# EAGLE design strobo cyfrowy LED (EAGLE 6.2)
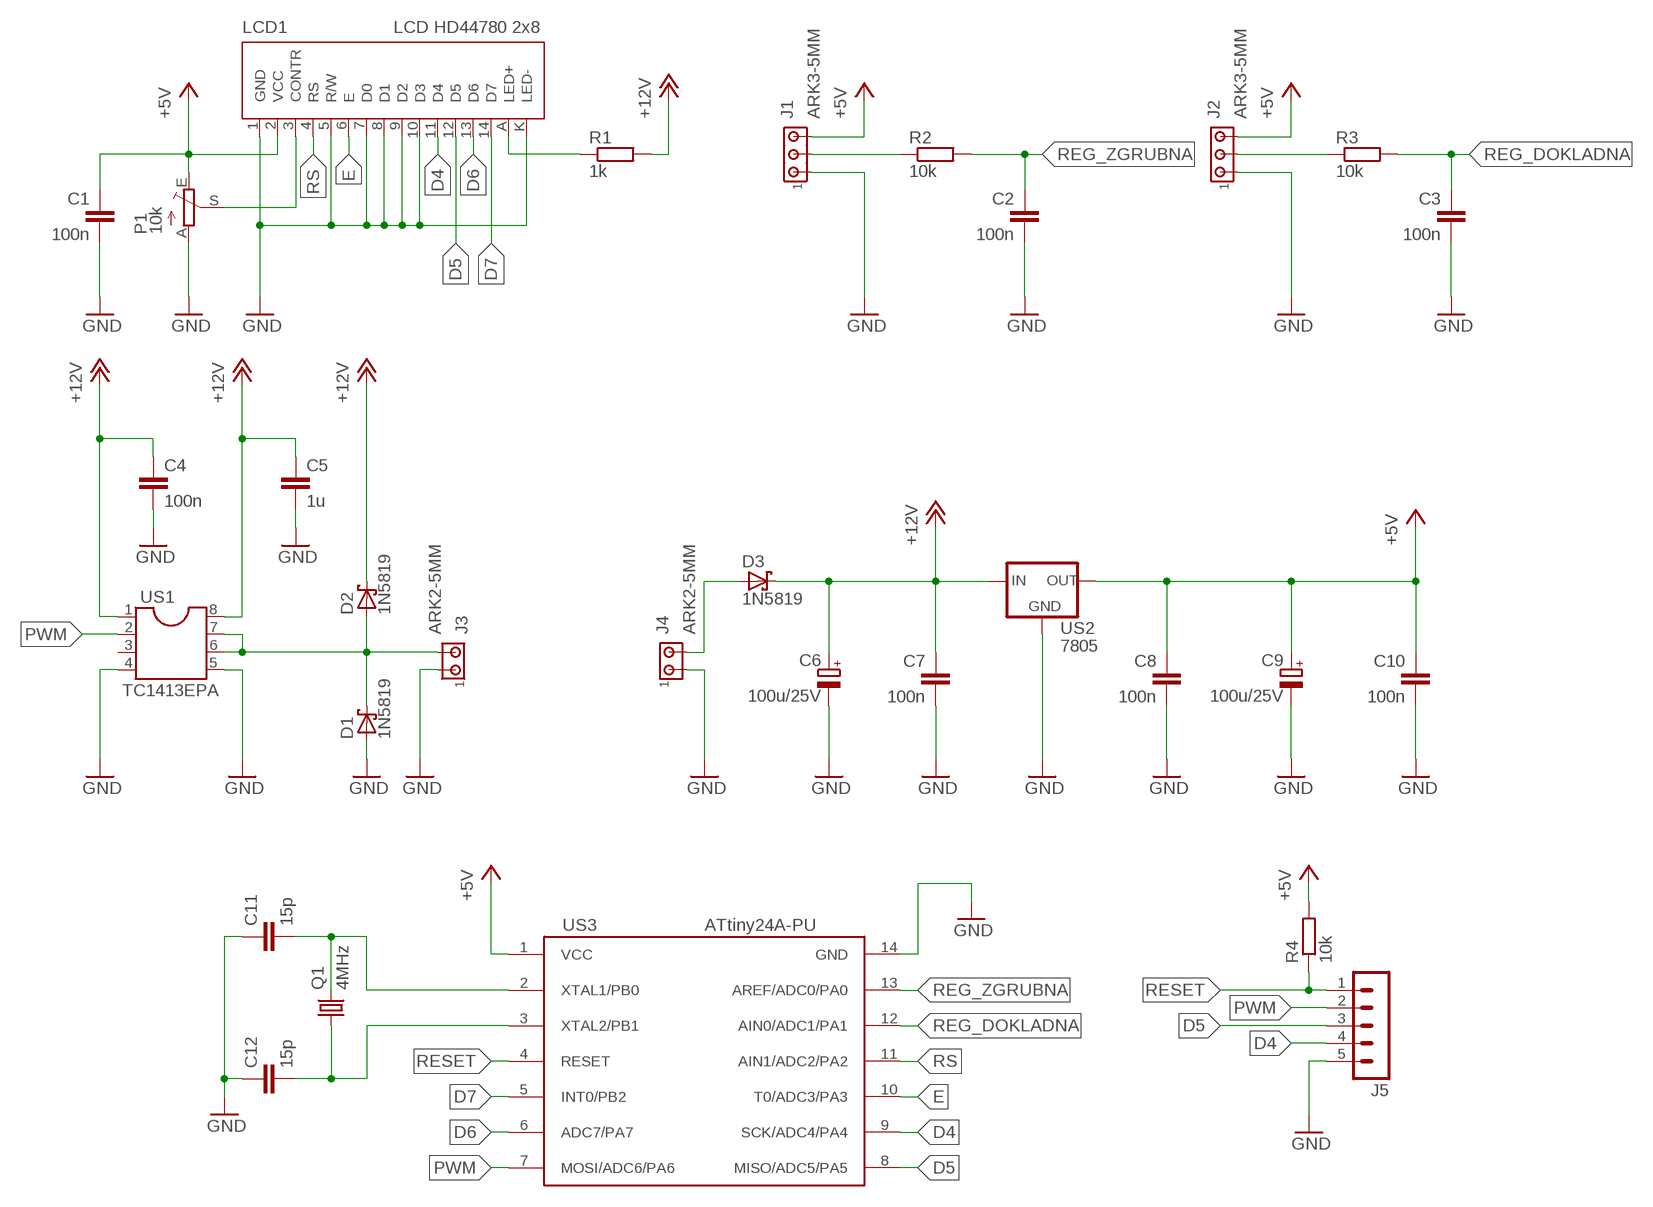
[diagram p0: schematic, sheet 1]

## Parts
C1  100n  C-EU050-025X075  [C050-025X075]
C2  100n  C-EU050-025X075  [C050-025X075]
C3  100n  C-EU050-025X075  [C050-025X075]
C4  100n  C-EU050-025X075  [C050-025X075]
C5  1u  C-EU050-055X075  [C050-055X075]
C6  100u/25V  CPOL-EUTT2D6L  [TT2D6L]
C7  100n  C-EU050-025X075  [C050-025X075]
C8  100n  C-EU050-025X075  [C050-025X075]
C9  100u/25V  CPOL-EUTT2D6L  [TT2D6L]
C10  100n  C-EU050-025X075  [C050-025X075]
C11  15p  C-EU050-025X075  [C050-025X075]
C12  15p  C-EU050-025X075  [C050-025X075]
D1  1N5819  SCHOTTKY-DIODEF126Z12  [F126Z12]
D2  1N5819  SCHOTTKY-DIODEF126Z12  [F126Z12]
D3  1N5819  SCHOTTKY-DIODEF126Z12  [F126Z12]
J1  ARK3-5MM  [3PIN-5MM]
J2  ARK3-5MM  [3PIN-5MM]
J3  ARK2-5MM  [2PIN-5MM]
J4  ARK2-5MM  [2PIN-5MM]
J5  MA05-1  [MA05-1]
LCD1  LCD HD44780 2x8  LCD_ZLACZE-MINI  [LCD_HD44780_1X6_NAD-ELEMENTAMI_Z-PODSW]
P1  10k  TRIM_EU-CA6V  [CA6V]
Q1  4MHz  CRYSTALHC49S  [HC49/S]
R1  1k  R-EU_0207/7  [0207/7]
R2  10k  R-EU_0207/2V  [0207/2V]
R3  10k  R-EU_0207/2V  [0207/2V]
R4  10k  R-EU_0207/7  [0207/7]
US1  TC1413EPA  DIL8  [DIL08]
US2  7805  78XXS  [78XXS]
US3  ATtiny24A-PU  ATTINY24/44/84-PU  [DIL14]

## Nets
+5V: C1.1 C8.1 C9.+ C10.1 J1.P$3 J2.P$3 LCD1.2(VCC) P1.E R4.2 US2.OUT US3.1(VCC)
+12V: C4.1 C5.1 C6.+ C7.1 D2.C D3.C R1.2 US1.1 US1.8 US2.IN
D4: J5.4 LCD1.11(D4) US3.9(SCK/ADC4/PA4)
D5: J5.3 LCD1.12(D5) US3.8(MISO/ADC5/PA5)
D6: LCD1.13(D6) US3.6(ADC7/PA7)
D7: LCD1.14(D7) US3.5(INT0/PB2)
E: LCD1.6(E) US3.10(T0/ADC3/PA3)
GND: C1.2 C2.2 C3.2 C4.2 C5.2 C6.- C7.2 C8.2 C9.- C10.2 C11.1 C12.1 D1.A J1.P$1 J2.P$1 J3.P$1 J4.P$1 J5.5 LCD1.1(GND) LCD1.5(R/W) LCD1.7(D0) LCD1.8(D1) LCD1.9(D2) LCD1.10(D3) LCD1.K(LED-) P1.A US1.4 US1.5 US2.GND US3.14(GND)
N$1: LCD1.3(CONTR) P1.S
N$2: C12.2 Q1.1 US3.3(XTAL2/PB1)
N$3: C11.2 Q1.2 US3.2(XTAL1/PB0)
N$4: J1.P$2 R2.1
N$5: LCD1.A(LED+) R1.1
N$6: J2.P$2 R3.1
N$7: D1.C D2.A J3.P$2 US1.6 US1.7
N$8: D3.A J4.P$2
PWM: J5.2 US1.2 US3.7(MOSI/ADC6/PA6)
REG_DOKLADNA: C3.1 R3.2 US3.12(AIN0/ADC1/PA1)
REG_ZGRUBNA: C2.1 R2.2 US3.13(AREF/ADC0/PA0)
RESET: J5.1 R4.1 US3.4(RESET)
RS: LCD1.4(RS) US3.11(AIN1/ADC2/PA2)
Unconnected: US1.3

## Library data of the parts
C1-C5 C7 C8 C10-C12 = rcl:C-EU: CAPACITOR, European symbol
C6 C9 = rcl:CPOL-EU: POLARIZED CAPACITOR, European symbol
D1-D3 = diode:SCHOTTKY-DIODE: Schottky Diode
J1 J2 = zlacza_futrzak:ARK3: ARK 3 Raster 5mm i 3,5mm
J3 J4 = zlacza_futrzak:ARK2: ARK 2
J5 = zlacza_futrzak:MA05-1: PIN HEADER; OC_FARNELL: unknown; OC_NEWARK: unknown
LCD1 = inne_futrzak:LCD_ZLACZE
P1 = pot:TRIM_EU-: POTENTIOMETER
Q1 = crystal:CRYSTAL: CRYSTAL; OC_FARNELL: 1667008; OC_NEWARK: unknown
R1-R4 = rcl:R-EU_: RESISTOR, European symbol
US1 = ic-package:DIL8: Dual In Line / Socket
US2 = v-reg:78XXS: VOLTAGE REGULATOR
US3 = scalaki_futrzak:ATTINY24/44/84

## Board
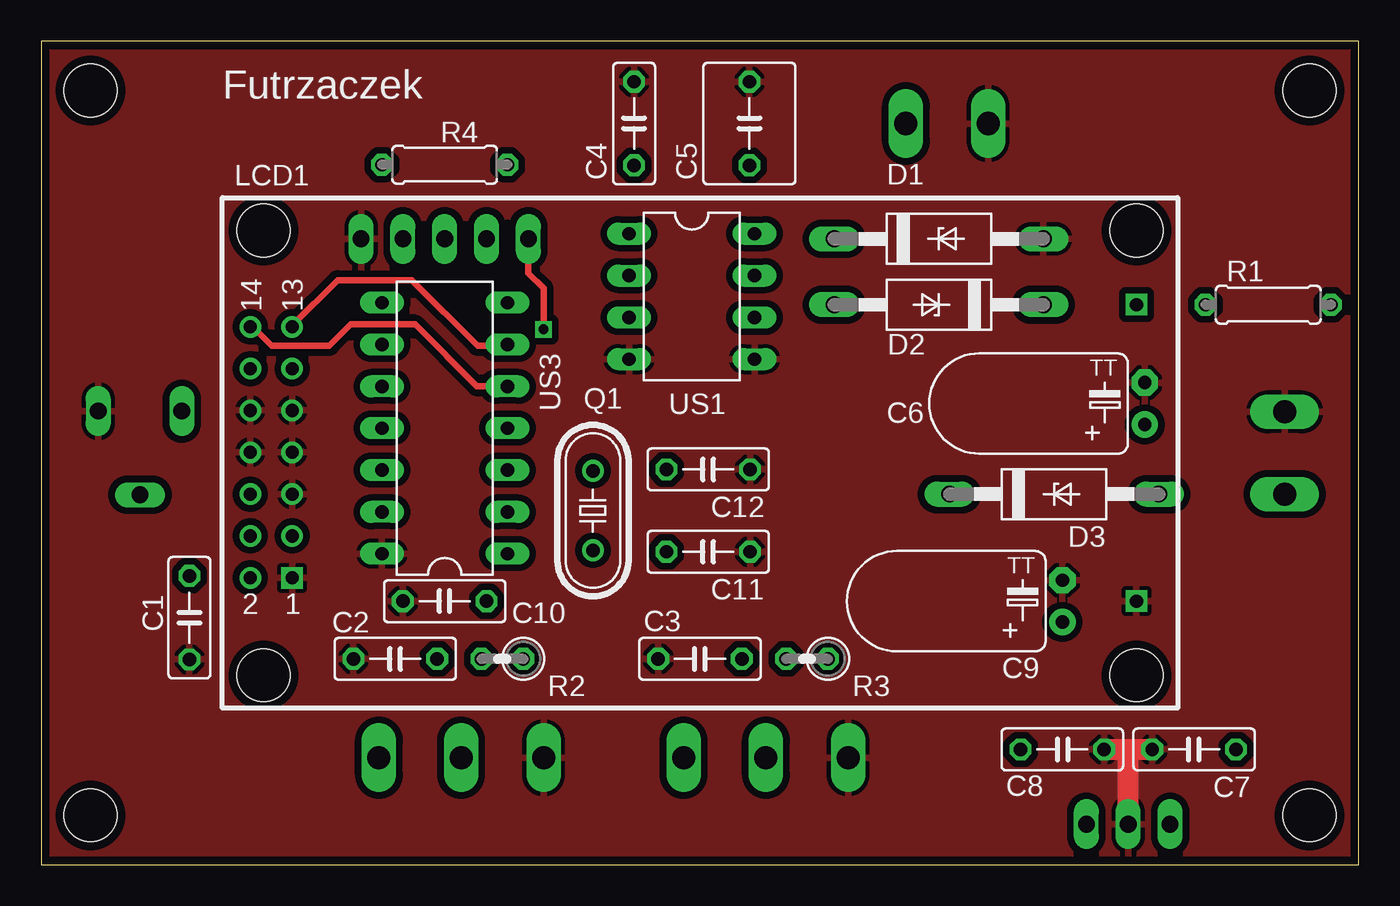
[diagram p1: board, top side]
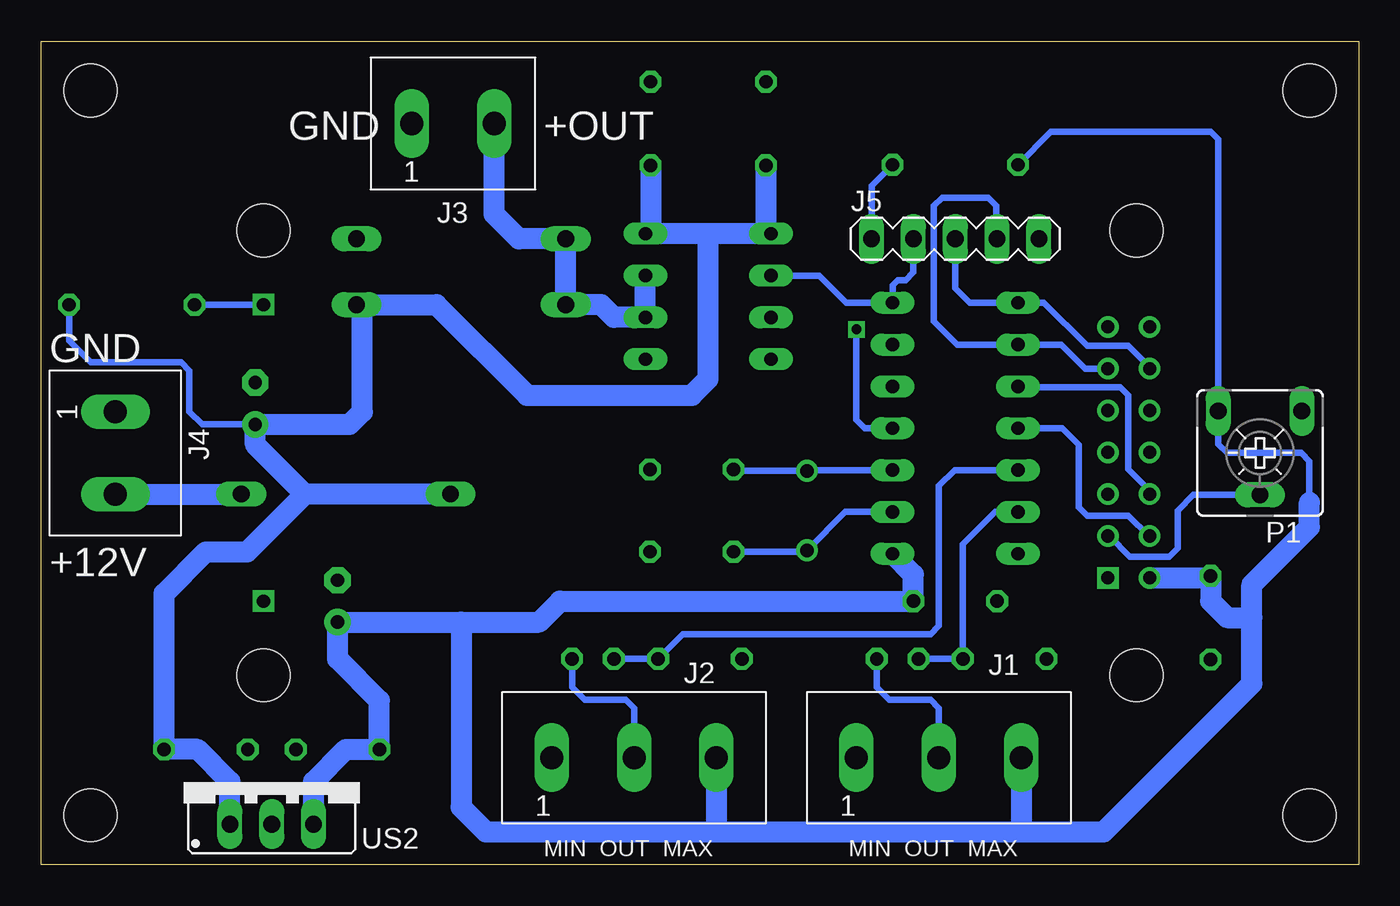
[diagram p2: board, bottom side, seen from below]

Size 80 x 50 mm. Coordinates in mm from the lower left corner, seen from the top.
Outline: 0,0 80,0 80,50 0,50 0,0
Copper layers (1*16): Top 0.035mm / dielectric 1.5mm / Bottom 0.035mm
Design rules: minimum track width 10mil, minimum drill 23mil, track to track 8mil, track to pad 8mil, pad to pad 8mil, via to via 8mil, smd to smd 8mil, copper to edge 20mil, drill to drill 8mil, minimum pad ring 10mil, minimum via ring 8mil, stop-mask expansion 4mil, vias tented up to drill 0mil, thermal gap 10mil
Holes 3.2 mm at 3,3 3,47 77,3 77,47

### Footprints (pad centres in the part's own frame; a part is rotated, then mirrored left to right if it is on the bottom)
C050-025X075 = drill 0.813 octagon: 1 -2.54,0; 2 2.54,0
C050-055X075 = drill 0.813 octagon: 1 -2.54,0; 2 2.54,0
TT2D6L = drill 0.813 pad 1.6: + -1.27,0 | drill 0.813 pad 1.6 octagon: - 1.27,0
F126Z12 = drill 1.016 long: A 6.35,0; C -6.35,0
3PIN-5MM = drill 1.4 long: P$1 -5,0; P$2 0,0; P$3 5,0
2PIN-5MM = drill 1.4 long: P$1 -2.5,0; P$2 2.5,0
MA05-1 = drill 1.016 long: 1 -5.08,0; 2 -2.54,0; 3 0,0; 4 2.54,0; 5 5.08,0
LCD_HD44780_1X6_NAD-ELEMENTAMI_Z-PODSW = drill 0.8 square: 1 1.74,5.92; A 53,22.5; K 53,4.5 | drill 0.8: 2 -0.8,5.92; 3 1.74,8.46; 4 -0.8,8.46; 5 1.74,11; 6 -0.8,11; 7 1.74,13.54; 8 -0.8,13.54; 9 1.74,16.08; 10 -0.8,16.08; 11 1.74,18.62; 12 -0.8,18.62; 13 1.74,21.16; 14 -0.8,21.16 | hole 3.2: 0,0; 0,27; 53,0; 53,27
CA6V = drill 1.016 long: A -2.54,-2.54; E 2.54,-2.54; S 0,2.54
HC49/S = drill 0.813: 1 -2.413,0; 2 2.413,0
0207/7 = drill 0.813 octagon: 1 -3.81,0; 2 3.81,0
0207/2V = drill 0.813 octagon: 1 -1.27,0; 2 1.27,0
DIL08 = drill 0.813 long: 1 -3.81,-3.81; 2 -1.27,-3.81; 3 1.27,-3.81; 4 3.81,-3.81; 5 3.81,3.81; 6 1.27,3.81; 7 -1.27,3.81; 8 -3.81,3.81
78XXS = drill 1.016 long: GND 0,-2.54; IN -2.54,-2.54; OUT 2.54,-2.54
DIL14 = drill 0.813 long: 1 -7.62,-3.81; 2 -5.08,-3.81; 3 -2.54,-3.81; 4 0,-3.81; 5 2.54,-3.81; 6 5.08,-3.81; 7 7.62,-3.81; 8 7.62,3.81; 9 5.08,3.81; 10 2.54,3.81; 11 0,3.81; 12 -2.54,3.81; 13 -5.08,3.81; 14 -7.62,3.81

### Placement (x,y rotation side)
C1  9,15 270 top
C2  21.5,12.5 180 top
C3  40,12.5 180 top
C4  36,45 90 top
C5  43,45 90 top
C6  67,28 90 top
C7  70,7 180 top
C8  62,7 0 top
C9  62,16 90 top
C10  24.5,16 180 top
C11  40.5,19 180 top
C12  40.5,24 180 top
D1  54.5,38 0 top
D2  54.5,34 180 top
D3  61.5,22.5 0 top
J1  25.5,6.5 0 bottom
J2  44,6.5 0 bottom
J3  55,45 0 bottom
J4  75.5,25 270 bottom
J5  24.5,38 0 bottom
LCD1  13.5,11.5 0 top
P1  6,25 180 bottom
Q1  33.5,21.5 270 top
R1  74.5,34 0 top
R2  28,12.5 180 top
R3  46.5,12.5 180 top
R4  24.5,42.5 180 top
US1  39.5,34.5 270 top
US2  66,5 0 bottom
US3  24.5,26.5 90 top

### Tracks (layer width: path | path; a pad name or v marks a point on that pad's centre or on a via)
+5V
  Bottom 0.406: R4.2 18.69,44.5 9,44.5 8.54,44.04 P1.E 8.54,25.54 8,25 3.5,25 3,24.5 3,22
  Bottom 1.27: US2.OUT 63.46,5.04 61.5,7 C8.1 59.46,9.96 62,12.5 C9.+ 54.5,14.73 | US3.1 27.04,17.61 C10.1 48.5,16 49.77,14.73 54.5,14.73 | 54.5,14.73 54.5,3.5 53,2 39,2 | 39,2 20.5,2 | 20.5,2 15.5,2 6.5,11 6.5,15 | 6.5,15 6.5,17 3,20.5 3,22 | LCD1.2 9.12,17.42 C1.1 9,16 8,15 6.5,15 | J1.P$3 20.5,2 | J2.P$3 39,2
+12V
  Bottom 0.406: C6.+ 70.23,26.73 71,27.5 71,30 71.5,30.5 77,30.5 78.31,31.81 R1.2
  Bottom 1.27: US1.1 36,38.31 | 36,38.31 39.5,38.31 | 39.5,38.31 US1.8 43,38.31 C5.1 | C4.1 36,38.31 | 39.5,38.31 39.5,29.5 40.5,28.5 50.5,28.5 56,34 D2.C 60.5,33.65 60.5,27.5 61.27,26.73 C6.+ 67,25.5 64,22.5 | D3.C 64,22.5 | US2.IN 68.54,5.04 70.5,7 C7.1 72.54,16.46 70,19 67.5,19 64,22.5
D4
  Bottom 0.406: J5.4 22,38.04 22,40 22.5,40.5 25.3,40.5 25.8,40 25.8,33 24.38,31.58 US3.9 18.08,31.58 16.62,30.12 LCD1.11
D5
  Bottom 0.406: J5.3 24.5,35 23.62,34.12 US3.8 19.12,34.12 16.5,31.5 14,31.5 12.7,30.2 LCD1.12
D6
  Top 0.406: LCD1.13 15.24,32.74 18,35.5 22.5,35.5 26.5,31.5 28.23,31.5 US3.6
D7
  Top 0.406: LCD1.14 12.84,32.66 14,31.5 17.5,31.5 18.8,32.8 22.7,32.8 26.46,29.04 US3.5
E
  Bottom 0.406: LCD1.6 12.7,22.7 14,24 14,28.5 14.5,29 20.65,29 US3.10
GND
  Top 1.27: US2.GND 66,7 | C8.2 C7.2
  pour Top (isolate 0.406): 0,0 80,0 80,50 0,50
N$1
  Bottom 0.406: LCD1.3 15.16,19.96 13.9,18.7 11.5,18.7 11,19.2 11,21.5 10.04,22.46 P1.S
N$2
  Bottom 0.406: US3.3 33.45,23.96 Q1.1 37.87,23.91 C12.2
N$3
  Bottom 0.406: US3.2 31.17,21.42 Q1.2 33.59,19 C11.2
N$4
  Bottom 0.406: J1.P$2 25.5,9.5 26,10 28.5,10 29.27,10.77 R2.1
N$5
  Bottom 0.406: LCD1.A R1.1
N$6
  Bottom 0.406: J2.P$2 44,9.5 44.5,10 47,10 47.77,10.77 R3.1
N$7
  Bottom 1.27: US1.7 US1.6 45.23,33.23 46,34 D2.A D1.C 51,38 52.5,39.5 J3.P$2
N$8
  Bottom 1.27: J4.P$2 D3.A
PWM
  Bottom 0.406: US1.2 32.77,35.77 31.12,34.12 US3.7 28.31,35.19 28,35.5 27.5,35.5 27.04,35.96 J5.2
REG_DOKLADNA
  Bottom 0.406: R3.2 C3.1 41.04,14 26,14 25.5,14.5 25.5,23 24.54,23.96 US3.12
REG_ZGRUBNA
  Bottom 0.406: R2.2 C2.1 24.04,19.46 22.08,21.42 US3.13
RESET  (via drill 0.6)
  Top 0.406: v30.5,32.5 30.5,35 29.58,35.92 J5.1
  Bottom 0.406: US3.4 30,26.5 30.5,27 v30.5,32.5 | J5.1 29.58,41.23 R4.1
RS
  Bottom 0.406: LCD1.4 12.76,19.96 14,21.2 16.5,21.2 17,21.7 17,25.5 18,26.5 US3.11

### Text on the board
tPlace: Futrzaczek
bPlace: +OUT | GND | GND | +12V | MIN OUT MAX | MIN OUT MAX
